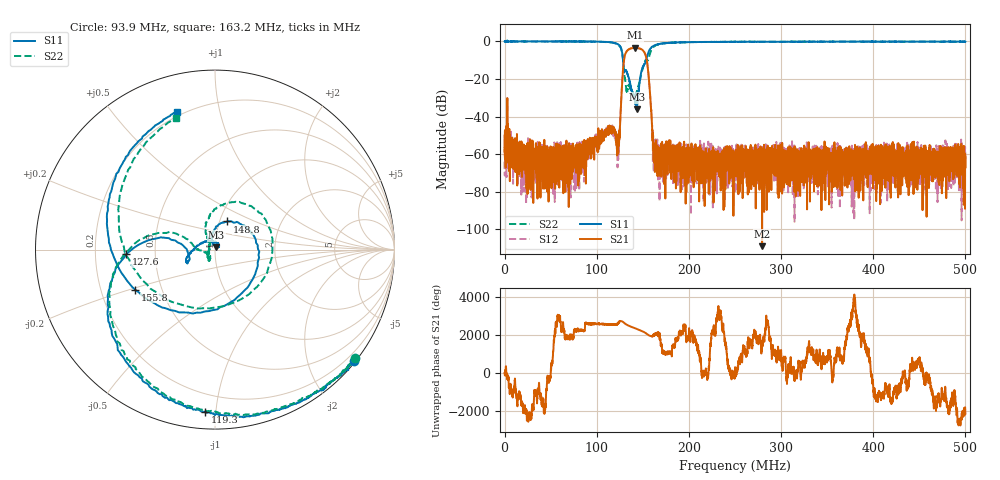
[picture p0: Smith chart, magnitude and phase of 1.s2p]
#  HZ  S  DB  R  50.00
! Rohde & Schwarz Vector Network Analyzer
! Rohde-Schwarz,ZNL6-2Port,1323001206101378,1.50.1.34-21.10.1.104
! Created: UTC 7/18/2023, 1:57:25 AM
! freq[Hz]  db:S11  ang:S11  db:S21  ang:S21  db:S12  ang:S12  db:S22  ang:S22
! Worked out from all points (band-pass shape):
!   5001 points, 5 kHz to 500 MHz, reference 50 ohm
!   highest |S21| = -3.38 dB at 141.6 MHz (marker M1); lowest = -109.1 dB at 279.4 MHz (marker M2)
!   |S21| within 3 dB of the highest: 131.2 MHz to 152.3 MHz (21.09 MHz wide, 14.9 % of centre)
!   lowest |S11| = -36.3 dB at 143.3 MHz (marker M3), VSWR 1.03, Z = 50.7 + j1.39 ohm
!   |S11| at or under -10 dB: 128.5 MHz to 153.6 MHz (25.11 MHz wide, 17.8 % of centre)
!   |S22| runs from -30.4 to 0.5 dB; largest |S21 - S12| = 0.048
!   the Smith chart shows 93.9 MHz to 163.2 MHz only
!   S11 on the Smith chart (normalised r, x): 93.9 MHz: 0.04, -2.84; 119.3 MHz: 0.09, -0.94; 127.6 MHz: 0.34, -0.02; 148.8 MHz: 1.09, +0.35; 155.8 MHz: 0.35, -0.21; 163.2 MHz: 0.18, +0.75
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5000  -0.01 -0.1  -58.69 -22.5  -64.18 -157.4  -0.03 -0.0
5004950  -0.03 -1.1  -50.64 21.5  -59.07 58.4  0.03 -1.9
4.690453e7  -0.02 -12.9  -68.97 107.1  -56.75 34.6  -0.03 -12.9
8.340417e7  -0.03 -29.9  -66.03 37.9  -55.10 78.3  -0.06 -29.2
9.390406e7  -0.07 -38.7  -54.74 50.0  -59.69 63.4  -0.12 -37.7
1.193038e8  -0.85 -93.5  -48.08 9.8  -48.96 19.0  -0.89 -91.7
1.235038e8  -1.66 -120.5  -55.86 98.8  -51.32 102.7  -1.77 -119.9
1.276037e8  -6.09 -177.0  -21.55 173.0  -21.79 173.4  -6.10 -178.1
1.334037e8  -17.19 -173.8  -4.70 -25.3  -4.75 -25.6  -25.38 -122.1
1.371036e8  -24.51 131.3  -3.71 -105.6  -3.69 -106.1  -25.01 -141.3
1.416036e8  -32.08 35.7  -3.38 171.0  -3.40 170.4  -29.02 155.9
1.433036e8  -36.27 63.0  -3.44 139.9  -3.49 139.7  -26.81 131.8
1.488035e8  -15.32 66.1  -4.25 32.2  -4.29 31.8  -16.38 109.3
1.558034e8  -6.06 -153.4  -15.93 -175.7  -15.89 -176.2  -9.89 -83.5
1.632034e8  -1.99 105.5  -57.33 164.2  -56.47 -126.2  -2.35 106.4
1.667033e8  -1.47 86.6  -68.26 -48.9  -63.87 -135.3  -1.64 85.3
1.901031e8  -0.47 37.9  -62.26 3.7  -61.43 55.4  -0.48 36.8
2.500025e8  -0.25 9.4  -64.96 153.2  -71.21 -118.1  -0.21 8.5
2.794022e8  -0.15 2.6  -109.09 -28.1  -68.09 1.8  -0.16 3.5
3.334017e8  -0.18 -4.1  -60.94 91.8  -60.77 165.0  -0.14 -4.8
4.167008e8  -0.16 -13.0  -74.35 18.2  -58.07 20.7  -0.13 -13.0
5e8  -0.10 -19.9  -61.78 -0.3  -62.64 -90.4  -0.14 -19.5
